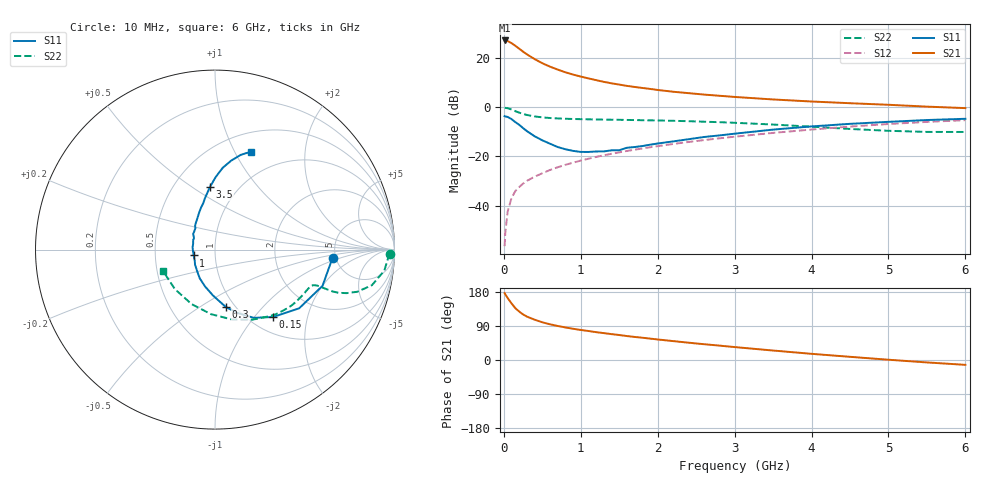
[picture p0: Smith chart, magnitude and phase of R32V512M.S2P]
! SIEMENS Small Signal Semiconductors
! BFR181
! Si NPN RF Bipolar Junction Transistor in SOT23
! VCE = 2.5 V  IC = 12 mA
! Common Emitter S-Parameters:  May  1996
# GHz  S  MA  R  50
!  f  S11  S21  S12  S22
! GHz  MAG  ANG  MAG  ANG  MAG  ANG  MAG  ANG
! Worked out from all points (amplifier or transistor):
!   36 points, 10 MHz to 6 GHz, reference 50 ohm
!   highest |S21| = 27.1 dB at 10 MHz (marker M1)
!   |S21| within 3 dB of that: start of sweep to 185 MHz
!   unconditionally stable (mu >= 1): 609 MHz to 2.645 GHz
!   at 250 MHz: K = 0.69, MSG = 26.8 dB, |S12| = -31.1 dB
!   at 1.4 GHz: K = 1.09, MAG = 12.5 dB, |S12| = -19.0 dB
!   at 6 GHz: K = 0.86, MSG = 2.4 dB, |S12| = -5.3 dB
!   S11 on the Smith chart (normalised r, x): 10 MHz: 4.70, -0.76; 150 MHz: 1.26, -1.25; 300 MHz: 0.91, -0.65; 1 GHz: 0.79, -0.05; 3.5 GHz: 0.74, +0.59; 6 GHz: 0.71, +1.16
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0.01  0.6569 -4.0  22.61 176.5  0.0015 90.0  0.9728 -1.3
0.02  0.6469 -7.4  22.46 173.0  0.0029 80.1  0.9652 -2.9
0.05  0.6322 -18.6  21.96 163.6  0.0076 79.6  0.9506 -7.1
0.1  0.5718 -34.9  19.97 149.3  0.0143 75.3  0.8963 -12.8
0.15  0.4953 -49.3  17.58 136.6  0.0198 71.2  0.827 -16.5
0.2  0.4374 -60.4  15.37 127.8  0.0238 69.7  0.7725 -18.3
0.25  0.375 -70.4  13.39 120.3  0.028 68.2  0.7285 -19.3
0.3  0.3257 -79.3  11.8 114.5  0.0318 68.3  0.6929 -19.6
0.4  0.2561 -92.5  9.458 106.4  0.0387 68.3  0.6478 -19.5
0.5  0.2119 -105.4  7.796 99.5  0.0453 69.2  0.6198 -19.4
0.6  0.1808 -118.2  6.644 94.2  0.0529 70.3  0.601 -19.4
0.7  0.1548 -130.3  5.788 89.8  0.0601 70.9  0.5895 -19.7
0.8  0.1395 -142.9  5.1 85.9  0.0673 71.1  0.5806 -20.0
1  0.1231 -164.8  4.173 79.3  0.0821 71.6  0.5695 -21.4
1.1  0.123 -175.9  3.836 76.5  0.0896 71.6  0.5649 -22.3
1.3  0.1261 164.8  3.259 70.9  0.1054 71.1  0.5582 -24.2
1.6  0.1496 144.5  2.702 63.2  0.1288 70.1  0.5494 -27.7
2.2  0.2012 119.1  2.056 49.9  0.1784 66.9  0.5278 -36.2
3.5  0.3497 94.7  1.432 25.0  0.2995 56.1  0.4427 -61.9
4.5  0.4579 84.6  1.201 8.4  0.4025 44.5  0.3604 -93.5
5.5  0.547 74.8  1.024 -6.4  0.5013 30.8  0.3138 -135.2
6  0.5798 70.0  0.955 -12.8  0.544 23.3  0.3131 -157.4
